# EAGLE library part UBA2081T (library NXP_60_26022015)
Half-bridge driver IC The UBA2080(A) and UBA2081 are high voltage monolithic integrated circuits made using the latch-up free Silicon-On-Insulator (SOI) process. The circuit is designed for driving MOSFETs in a half-bridge configuration. AAL Eindhoven MK
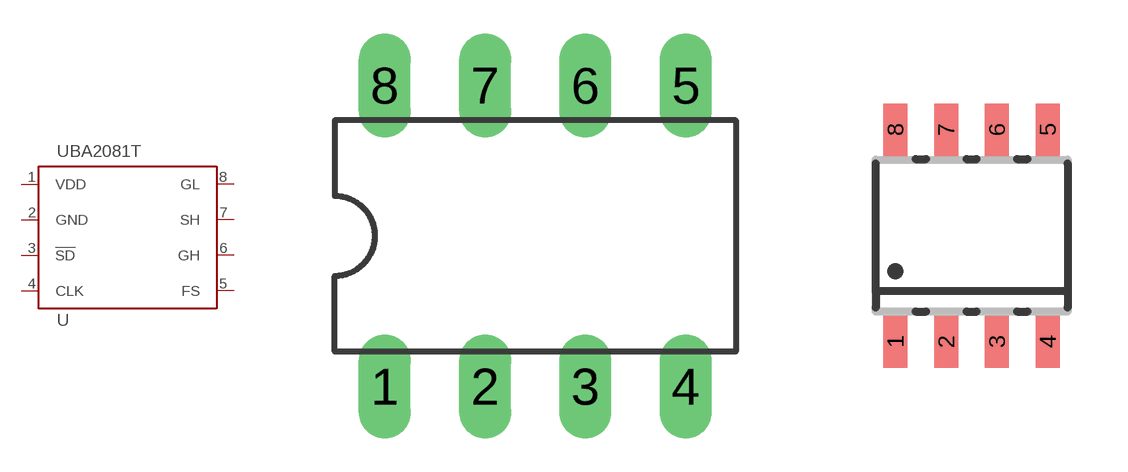
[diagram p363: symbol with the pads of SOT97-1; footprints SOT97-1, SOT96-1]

Designator prefix U

## UBA2081TP  [SOT97-1]
1  VDD  pwr
2  GND  pwr
3  !SD  in
4  CLK  in
5  FS  pas
6  GH  pas
7  SH  out
8  GL  out

## UBA2081TT  [SOT96-1]
Pads as for SOT97-1

## Footprint SOT97-1 (pad centres in mm)
Dual In Line Package
drill 0.813 long: 1 -3.81,-3.81; 2 -1.27,-3.81; 3 1.27,-3.81; 4 3.81,-3.81; 5 3.81,3.81; 6 1.27,3.81; 7 -1.27,3.81; 8 -3.81,3.81

## Footprint SOT96-1 (pad centres in mm)
SOT96-1 SO8: plastic small outline package; 8 leads; body width 3.9 mm JEDEC: MS-012 IEC: 076E03
smd 0.6 x 1.3: 1 -1.905,-2.65; 2 -0.635,-2.65; 3 0.635,-2.65; 4 1.905,-2.65; 5 1.905,2.65; 6 0.635,2.65; 7 -0.635,2.65; 8 -1.905,2.65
